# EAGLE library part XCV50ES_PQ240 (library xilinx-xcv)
xcv50es_pq240 edit this description Auto generated by make-symbol-device-package-bsdl.ulp Rev. 26 Source: xcv50es_pq240.bsd
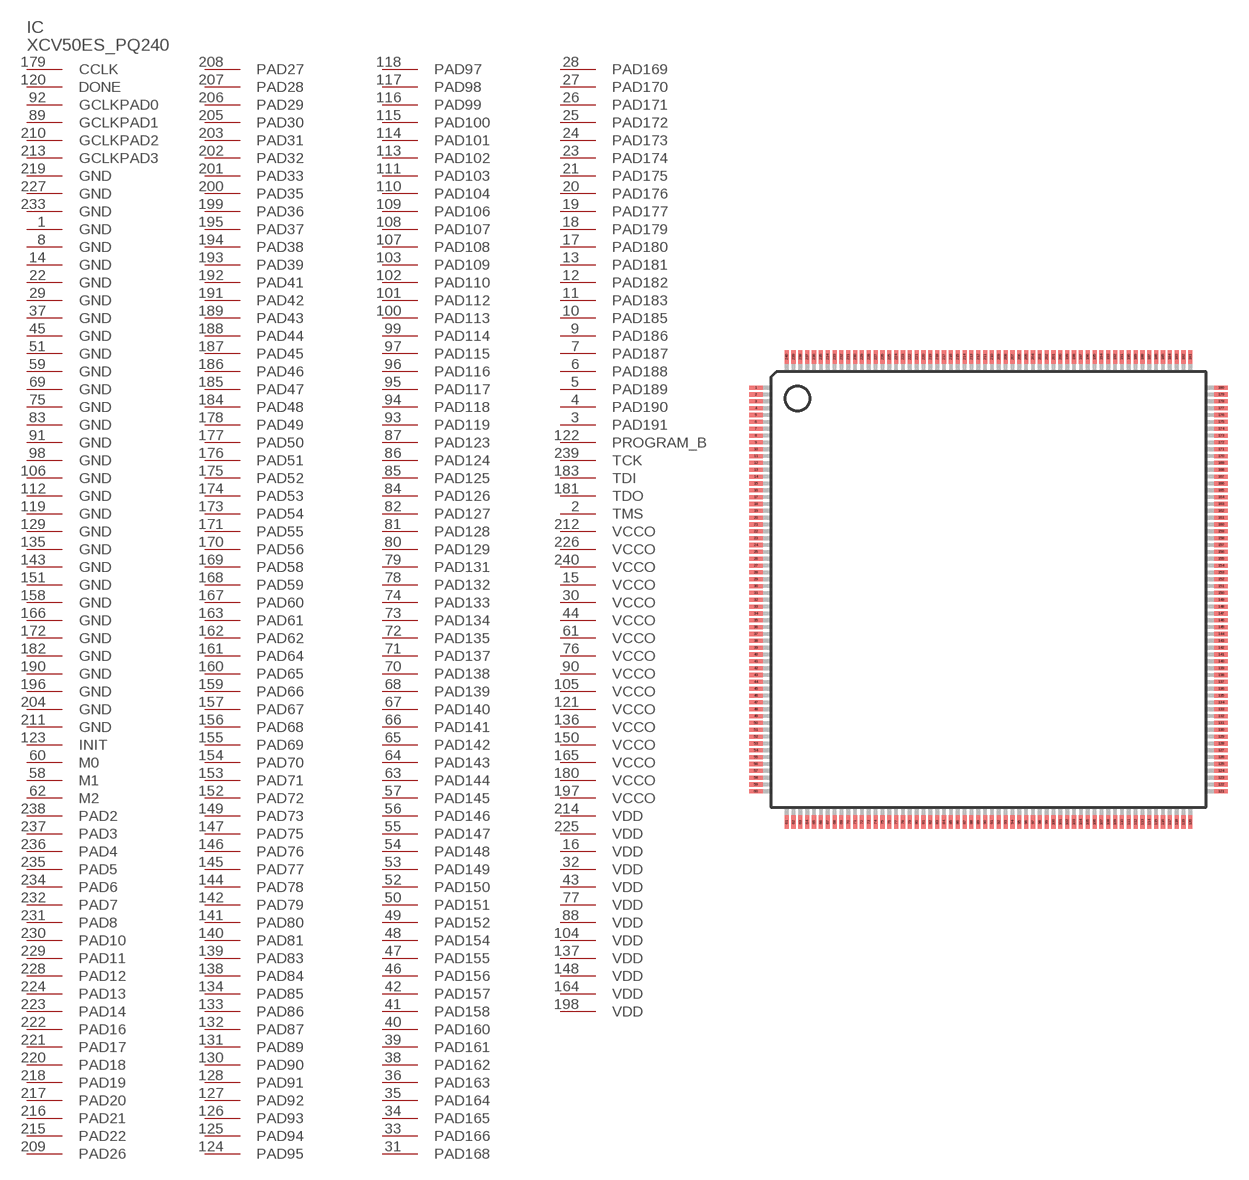
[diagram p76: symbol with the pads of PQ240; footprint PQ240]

Designator prefix IC

## XCV50ES_PQ240 (OC_FARNELL: unknown; OC_NEWARK: unknown)  [PQ240]
1  GND  pwr
2  TMS  in
3  PAD191
4  PAD190
5  PAD189
6  PAD188
7  PAD187
8  GND  pwr
9  PAD186
10  PAD185
11  PAD183
12  PAD182
13  PAD181
14  GND  pwr
15  VCCO  pwr
16  VDD  pwr
17  PAD180
18  PAD179
19  PAD177
20  PAD176
21  PAD175
22  GND  pwr
23  PAD174
24  PAD173
25  PAD172
26  PAD171
27  PAD170
28  PAD169
29  GND  pwr
30  VCCO  pwr
31  PAD168
32  VDD  pwr
33  PAD166
34  PAD165
35  PAD164
36  PAD163
37  GND  pwr
38  PAD162
39  PAD161
40  PAD160
41  PAD158
42  PAD157
43  VDD  pwr
44  VCCO  pwr
45  GND  pwr
46  PAD156
47  PAD155
48  PAD154
49  PAD152
50  PAD151
51  GND  pwr
52  PAD150
53  PAD149
54  PAD148
55  PAD147
56  PAD146
57  PAD145
58  M1  in
59  GND  pwr
60  M0  in
61  VCCO  pwr
62  M2  in
63  PAD144
64  PAD143
65  PAD142
66  PAD141
67  PAD140
68  PAD139
69  GND  pwr
70  PAD138
71  PAD137
72  PAD135
73  PAD134
74  PAD133
75  GND  pwr
76  VCCO  pwr
77  VDD  pwr
78  PAD132
79  PAD131
80  PAD129
81  PAD128
82  PAD127
83  GND  pwr
84  PAD126
85  PAD125
86  PAD124
87  PAD123
88  VDD  pwr
89  GCLKPAD1  in
90  VCCO  pwr
91  GND  pwr
92  GCLKPAD0  in
93  PAD119
94  PAD118
95  PAD117
96  PAD116
97  PAD115
98  GND  pwr
99  PAD114
100  PAD113
101  PAD112
102  PAD110
103  PAD109
104  VDD  pwr
105  VCCO  pwr
106  GND  pwr
107  PAD108
108  PAD107
109  PAD106
110  PAD104
111  PAD103
112  GND  pwr
113  PAD102
114  PAD101
115  PAD100
116  PAD99
117  PAD98
118  PAD97
119  GND  pwr
120  DONE
121  VCCO  pwr
122  PROGRAM_B  in
123  INIT
124  PAD95
125  PAD94
126  PAD93
127  PAD92
128  PAD91
129  GND  pwr
130  PAD90
131  PAD89
132  PAD87
133  PAD86
134  PAD85
135  GND  pwr
136  VCCO  pwr
137  VDD  pwr
138  PAD84
139  PAD83
140  PAD81
141  PAD80
142  PAD79
143  GND  pwr
144  PAD78
145  PAD77
146  PAD76
147  PAD75
148  VDD  pwr
149  PAD73
150  VCCO  pwr
151  GND  pwr
152  PAD72
153  PAD71
154  PAD70
155  PAD69
156  PAD68
157  PAD67
158  GND  pwr
159  PAD66
160  PAD65
161  PAD64
162  PAD62
163  PAD61
164  VDD  pwr
165  VCCO  pwr
166  GND  pwr
167  PAD60
168  PAD59
169  PAD58
170  PAD56
171  PAD55
172  GND  pwr
173  PAD54
174  PAD53
175  PAD52
176  PAD51
177  PAD50
178  PAD49
179  CCLK
180  VCCO  pwr
181  TDO  out
182  GND  pwr
183  TDI  in
184  PAD48
185  PAD47
186  PAD46
187  PAD45
188  PAD44
189  PAD43
190  GND  pwr
191  PAD42
192  PAD41
193  PAD39
194  PAD38
195  PAD37
196  GND  pwr
197  VCCO  pwr
198  VDD  pwr
199  PAD36
200  PAD35
201  PAD33
202  PAD32
203  PAD31
204  GND  pwr
205  PAD30
206  PAD29
207  PAD28
208  PAD27
209  PAD26
210  GCLKPAD2  in
211  GND  pwr
212  VCCO  pwr
213  GCLKPAD3  in
214  VDD  pwr
215  PAD22
216  PAD21
217  PAD20
218  PAD19
219  GND  pwr
220  PAD18
221  PAD17
222  PAD16
223  PAD14
224  PAD13
225  VDD  pwr
226  VCCO  pwr
227  GND  pwr
228  PAD12
229  PAD11
230  PAD10
231  PAD8
232  PAD7
233  GND  pwr
234  PAD6
235  PAD5
236  PAD4
237  PAD3
238  PAD2
239  TCK  in
240  VCCO  pwr

## Footprint PQ240 (pad centres in mm)
PQ240 Auto generated by make-symbol-device-package-bsdl.ulp Rev. 26
smd 1 x 0.3: 1 -17,14.75; 2 -17,14.25; 3 -17,13.75; 4 -17,13.25; 5 -17,12.75; 6 -17,12.25; 7 -17,11.75; 8 -17,11.25; 9 -17,10.75; 10 -17,10.25; 11 -17,9.75; 12 -17,9.25; 13 -17,8.75; 14 -17,8.25; 15 -17,7.75; 16 -17,7.25; 17 -17,6.75; 18 -17,6.25; 19 -17,5.75; 20 -17,5.25; 21 -17,4.75; 22 -17,4.25; 23 -17,3.75; 24 -17,3.25; 25 -17,2.75; 26 -17,2.25; 27 -17,1.75; 28 -17,1.25; 29 -17,0.75; 30 -17,0.25; 31 -17,-0.25; 32 -17,-0.75; 33 -17,-1.25; 34 -17,-1.75; 35 -17,-2.25; 36 -17,-2.75; 37 -17,-3.25; 38 -17,-3.75; 39 -17,-4.25; 40 -17,-4.75; 41 -17,-5.25; 42 -17,-5.75; 43 -17,-6.25; 44 -17,-6.75; 45 -17,-7.25; 46 -17,-7.75; 47 -17,-8.25; 48 -17,-8.75; 49 -17,-9.25; 50 -17,-9.75; 51 -17,-10.25; 52 -17,-10.75; 53 -17,-11.25; 54 -17,-11.75; 55 -17,-12.25; 56 -17,-12.75; 57 -17,-13.25; 58 -17,-13.75; 59 -17,-14.25; 60 -17,-14.75; 121 17,-14.75; 122 17,-14.25; 123 17,-13.75; 124 17,-13.25; 125 17,-12.75; 126 17,-12.25; 127 17,-11.75; 128 17,-11.25; 129 17,-10.75; 130 17,-10.25; 131 17,-9.75; 132 17,-9.25; 133 17,-8.75; 134 17,-8.25; 135 17,-7.75; 136 17,-7.25; 137 17,-6.75; 138 17,-6.25; 139 17,-5.75; 140 17,-5.25; 141 17,-4.75; 142 17,-4.25; 143 17,-3.75; 144 17,-3.25; 145 17,-2.75; 146 17,-2.25; 147 17,-1.75; 148 17,-1.25; 149 17,-0.75; 150 17,-0.25; 151 17,0.25; 152 17,0.75; 153 17,1.25; 154 17,1.75; 155 17,2.25; 156 17,2.75; 157 17,3.25; 158 17,3.75; 159 17,4.25; 160 17,4.75; 161 17,5.25; 162 17,5.75; 163 17,6.25; 164 17,6.75; 165 17,7.25; 166 17,7.75; 167 17,8.25; 168 17,8.75; 169 17,9.25; 170 17,9.75; 171 17,10.25; 172 17,10.75; 173 17,11.25; 174 17,11.75; 175 17,12.25; 176 17,12.75; 177 17,13.25; 178 17,13.75; 179 17,14.25; 180 17,14.75
smd 0.3 x 1: 61 -14.75,-17; 62 -14.25,-17; 63 -13.75,-17; 64 -13.25,-17; 65 -12.75,-17; 66 -12.25,-17; 67 -11.75,-17; 68 -11.25,-17; 69 -10.75,-17; 70 -10.25,-17; 71 -9.75,-17; 72 -9.25,-17; 73 -8.75,-17; 74 -8.25,-17; 75 -7.75,-17; 76 -7.25,-17; 77 -6.75,-17; 78 -6.25,-17; 79 -5.75,-17; 80 -5.25,-17; 81 -4.75,-17; 82 -4.25,-17; 83 -3.75,-17; 84 -3.25,-17; 85 -2.75,-17; 86 -2.25,-17; 87 -1.75,-17; 88 -1.25,-17; 89 -0.75,-17; 90 -0.25,-17; 91 0.25,-17; 92 0.75,-17; 93 1.25,-17; 94 1.75,-17; 95 2.25,-17; 96 2.75,-17; 97 3.25,-17; 98 3.75,-17; 99 4.25,-17; 100 4.75,-17; 101 5.25,-17; 102 5.75,-17; 103 6.25,-17; 104 6.75,-17; 105 7.25,-17; 106 7.75,-17; 107 8.25,-17; 108 8.75,-17; 109 9.25,-17; 110 9.75,-17; 111 10.25,-17; 112 10.75,-17; 113 11.25,-17; 114 11.75,-17; 115 12.25,-17; 116 12.75,-17; 117 13.25,-17; 118 13.75,-17; 119 14.25,-17; 120 14.75,-17; 181 14.75,17; 182 14.25,17; 183 13.75,17; 184 13.25,17; 185 12.75,17; 186 12.25,17; 187 11.75,17; 188 11.25,17; 189 10.75,17; 190 10.25,17; 191 9.75,17; 192 9.25,17; 193 8.75,17; 194 8.25,17; 195 7.75,17; 196 7.25,17; 197 6.75,17; 198 6.25,17; 199 5.75,17; 200 5.25,17; 201 4.75,17; 202 4.25,17; 203 3.75,17; 204 3.25,17; 205 2.75,17; 206 2.25,17; 207 1.75,17; 208 1.25,17; 209 0.75,17; 210 0.25,17; 211 -0.25,17; 212 -0.75,17; 213 -1.25,17; 214 -1.75,17; 215 -2.25,17; 216 -2.75,17; 217 -3.25,17; 218 -3.75,17; 219 -4.25,17; 220 -4.75,17; 221 -5.25,17; 222 -5.75,17; 223 -6.25,17; 224 -6.75,17; 225 -7.25,17; 226 -7.75,17; 227 -8.25,17; 228 -8.75,17; 229 -9.25,17; 230 -9.75,17; 231 -10.25,17; 232 -10.75,17; 233 -11.25,17; 234 -11.75,17; 235 -12.25,17; 236 -12.75,17; 237 -13.25,17; 238 -13.75,17; 239 -14.25,17; 240 -14.75,17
